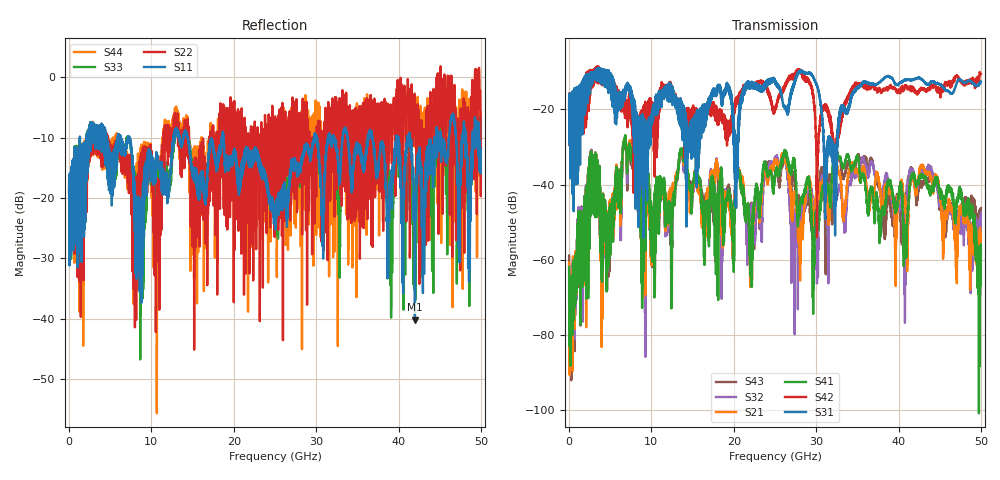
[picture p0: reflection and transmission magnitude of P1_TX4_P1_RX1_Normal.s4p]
!Keysight Technologies,N5225B,MY57041031,A.13.20.10
!Date: Friday, May 31, 2019 11:14:01
!Correction: S11(Full 4 Port(1,2,3,4))
!S12(Full 4 Port(1,2,3,4))
!S13(Full 4 Port(1,2,3,4))
!S14(Full 4 Port(1,2,3,4))
!S21(Full 4 Port(1,2,3,4))
!S22(Full 4 Port(1,2,3,4))
!S23(Full 4 Port(1,2,3,4))
!S24(Full 4 Port(1,2,3,4))
!S31(Full 4 Port(1,2,3,4))
!S32(Full 4 Port(1,2,3,4))
!S33(Full 4 Port(1,2,3,4))
!S34(Full 4 Port(1,2,3,4))
!S41(Full 4 Port(1,2,3,4))
!S42(Full 4 Port(1,2,3,4))
!S43(Full 4 Port(1,2,3,4))
!S44(Full 4 Port(1,2,3,4))
!S4P File: Measurements: <S11,S12,S13,S14>,
!<S21,S22,S23,S24>,
!<S31,S32,S33,S34>,
!<S41,S42,S43,S44>:
# Hz S  dB  R 50.0
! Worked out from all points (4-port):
!   5000 points, 10 MHz to 50 GHz, reference 50 ohm
!   strongest paths, dB at 10 MHz, 12.51 GHz, 25.01 GHz, 37.51 GHz, 50 GHz:
!     S31: -19.6, -17.6, -12.9, -13.0, -12.6
!     S42: -19.4, -14.7, -19.9, -15.1, -10.5
!     S41: -61.8, -56.4, -37.9, -45.7, -58.3
!     S21: -60.8, -44.1, -34.3, -37.8, -54.7
!     S32: -70.9, -44.5, -33.2, -39.0, -47.5
!     S43: -58.8, -55.9, -37.5, -40.3, -46.2
!   lowest |S11| = -40.2 dB at 41.99 GHz (marker M1), VSWR 1.02, Z = 50.9 - j0.302 ohm
!   |S11| at or under -10 dB: 7.336 GHz to 12.7 GHz (5.362 GHz wide, 53.5 % of centre); 14.41 GHz to 18.57 GHz (4.157 GHz wide, 25.2 % of centre); 18.74 GHz to 29.76 GHz (11.02 GHz wide, 45.4 % of centre)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
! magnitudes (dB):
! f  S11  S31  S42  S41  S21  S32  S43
! 10 MHz  -19.5  -19.6  -19.4  -61.8  -60.8  -70.9  -58.8
! 6.72 GHz  -11.9  -16.0  -18.7  -29.0  -28.8  -29.1  -29.6
! 20.59 GHz  -17.3  -26.2  -16.2  -36.3  -35.8  -35.7  -36.0
! 22.12 GHz  -12.7  -13.2  -13.9  -54.2  -58.4  -46.4  -45.7
! 32.24 GHz  -10.5  -35.7  -36.7  -31.3  -35.8  -43.8  -35.5
! 41.99 GHz  -40.2  -12.0  -14.9  -38.9  -41.0  -40.8  -40.9
! 50 GHz  -12.0  -12.6  -10.5  -58.3  -54.7  -47.5  -46.2
